|Texas Instruments Incorporated
|ADS890xB 20-Bit, High-Speed SAR ADCs With Integrated Reference Buffer, and
|Enhanced Performance Features
[IBIS Ver]   4.1
[File name]   ads890xb.ibs
[Date]   07/31/2018
[File Rev]   1.0
[Source]
| Texas Instruments Incorporated.
| Analog-eLab Design Center, HPA
| 12500 TI Blvd
| Dallas, TX -75243
[Notes]   Revision History:
| Rev 1.0: 07/31/2018
| - Initial version of the model
| - Model generated from simulations in SPECTRE
| - Warnings regarding combined Non-monotonicity of various models
|   have been reviewed and considered minor and can be ignored.
| - C_comp although listed in numerical order of value are
|   obtained from varying PVT conditions. For PVT conditions for
|   each specific value refer the buffer description under
|   respective [Model]. IBIS model user is responsible for using
|   appropriate C_comp to simulate for Signal Integrity.
[Disclaimer]
| This model is designed as an aid for customers of Texas Instruments.
| TI and its licensors and suppliers make no warranties, either expressed
| or implied, with respect to this  model, including the warranties of
| merchantability or fitness for a particular purpose. The model is
| provided solely on an "as is" basis. The entire risk as to its quality
| and performance is with the customer.
| This model is subject to change without notice. Texas Instruments
| Incorporated is not responsible for updating this model.
[Copyright]
(C) Copyright 2018 Texas Instruments Incorporated.All rights reserved.
|  Component ADS8900BRGER 24-pin VQFN - RGE package
|  Part # ADS8900BRGER
[Component]   ADS8900BRGER
[Manufacturer]  TI
[Package]   |24-pin VQFN - RGE package
|   typ   min   max
R_pkg   0.05   0.04   0.06
L_pkg   1.0nH   0.8nH   1.2nH
C_pkg   0.2pF   0.16pF   0.24pF
[Pin] signal_name model_name R_pin L_pin C_pin
1   CONVST   INPUT   NA   NA   NA
2   RSTZ   INPUT   NA   NA   NA
3   REFIN   NC   NA   NA   NA
4   REFM   NC   NA   NA   NA
5   REFBUFOUT   NC   NA   NA   NA
6   NC   NC   NA   NA   NA
7   REFBUFOUT   NC   NA   NA   NA
8   REFM   NC   NA   NA   NA
9   AINP   NC   NA   NA   NA
10   AINM   NC   NA   NA   NA
11   GND   GND   NA   NA   NA
12   RVDD   POWER   NA   NA   NA
13   DECAP   POWER   NA   NA   NA
14   DECAP   POWER   NA   NA   NA
15   GND   GND   NA   NA   NA
16   DVDD   POWER   NA   NA   NA
17   SDO-3   OUTPUT   NA   NA   NA
18   SDO-2   OUTPUT   NA   NA   NA
19   SDO-1   OUTPUT   NA   NA   NA
20   SDO-0   OUTPUT   NA   NA   NA
21   RVS   OUTPUT   NA   NA   NA
22   SDI   INPUT   NA   NA   NA
23   SCLK   INPUT   NA   NA   NA
24   CSZ   INPUT   NA   NA   NA
|  Component ADS8900BRGET 24-pin VQFN - RGE package
|  Part # ADS8900BRGET
[Component]   ADS8900BRGET
[Manufacturer]  TI
[Package]   |24-pin VQFN - RGE package
|   typ   min   max
R_pkg   0.05   0.04   0.06
L_pkg   1.0nH   0.8nH   1.2nH
C_pkg   0.2pF   0.16pF   0.24pF
[Pin] signal_name model_name R_pin L_pin C_pin
1   CONVST   INPUT   NA   NA   NA
2   RSTZ   INPUT   NA   NA   NA
3   REFIN   NC   NA   NA   NA
4   REFM   NC   NA   NA   NA
5   REFBUFOUT   NC   NA   NA   NA
6   NC   NC   NA   NA   NA
7   REFBUFOUT   NC   NA   NA   NA
8   REFM   NC   NA   NA   NA
9   AINP   NC   NA   NA   NA
10   AINM   NC   NA   NA   NA
11   GND   GND   NA   NA   NA
12   RVDD   POWER   NA   NA   NA
13   DECAP   POWER   NA   NA   NA
14   DECAP   POWER   NA   NA   NA
15   GND   GND   NA   NA   NA
16   DVDD   POWER   NA   NA   NA
17   SDO-3   OUTPUT   NA   NA   NA
18   SDO-2   OUTPUT   NA   NA   NA
19   SDO-1   OUTPUT   NA   NA   NA
20   SDO-0   OUTPUT   NA   NA   NA
21   RVS   OUTPUT   NA   NA   NA
22   SDI   INPUT   NA   NA   NA
23   SCLK   INPUT   NA   NA   NA
24   CSZ   INPUT   NA   NA   NA
|  Component ADS8902BRGER 24-pin VQFN - RGE package
|  Part # ADS8902BRGER
[Component]   ADS8902BRGER
[Manufacturer]  TI
[Package]   |24-pin VQFN - RGE package
|   typ   min   max
R_pkg   0.05   0.04   0.06
L_pkg   1.0nH   0.8nH   1.2nH
C_pkg   0.2pF   0.16pF   0.24pF
[Pin] signal_name model_name R_pin L_pin C_pin
1   CONVST   INPUT   NA   NA   NA
2   RSTZ   INPUT   NA   NA   NA
3   REFIN   NC   NA   NA   NA
4   REFM   NC   NA   NA   NA
5   REFBUFOUT   NC   NA   NA   NA
6   NC   NC   NA   NA   NA
7   REFBUFOUT   NC   NA   NA   NA
8   REFM   NC   NA   NA   NA
9   AINP   NC   NA   NA   NA
10   AINM   NC   NA   NA   NA
11   GND   GND   NA   NA   NA
12   RVDD   POWER   NA   NA   NA
13   DECAP   POWER   NA   NA   NA
14   DECAP   POWER   NA   NA   NA
15   GND   GND   NA   NA   NA
16   DVDD   POWER   NA   NA   NA
17   SDO-3   OUTPUT   NA   NA   NA
18   SDO-2   OUTPUT   NA   NA   NA
19   SDO-1   OUTPUT   NA   NA   NA
20   SDO-0   OUTPUT   NA   NA   NA
21   RVS   OUTPUT   NA   NA   NA
22   SDI   INPUT   NA   NA   NA
23   SCLK   INPUT   NA   NA   NA
24   CSZ   INPUT   NA   NA   NA
|  Component ADS8902BRGET 24-pin VQFN - RGE package
|  Part # ADS8902BRGET
[Component]   ADS8902BRGET
[Manufacturer]  TI
[Package]   |24-pin VQFN - RGE package
|   typ   min   max
R_pkg   0.05   0.04   0.06
L_pkg   1.0nH   0.8nH   1.2nH
C_pkg   0.2pF   0.16pF   0.24pF
[Pin] signal_name model_name R_pin L_pin C_pin
1   CONVST   INPUT   NA   NA   NA
2   RSTZ   INPUT   NA   NA   NA
3   REFIN   NC   NA   NA   NA
4   REFM   NC   NA   NA   NA
5   REFBUFOUT   NC   NA   NA   NA
6   NC   NC   NA   NA   NA
7   REFBUFOUT   NC   NA   NA   NA
8   REFM   NC   NA   NA   NA
9   AINP   NC   NA   NA   NA
10   AINM   NC   NA   NA   NA
11   GND   GND   NA   NA   NA
12   RVDD   POWER   NA   NA   NA
13   DECAP   POWER   NA   NA   NA
14   DECAP   POWER   NA   NA   NA
15   GND   GND   NA   NA   NA
16   DVDD   POWER   NA   NA   NA
17   SDO-3   OUTPUT   NA   NA   NA
18   SDO-2   OUTPUT   NA   NA   NA
19   SDO-1   OUTPUT   NA   NA   NA
20   SDO-0   OUTPUT   NA   NA   NA
21   RVS   OUTPUT   NA   NA   NA
22   SDI   INPUT   NA   NA   NA
23   SCLK   INPUT   NA   NA   NA
24   CSZ   INPUT   NA   NA   NA
|  Component ADS8904BRGER 24-pin VQFN - RGE package
|  Part # ADS8904BRGER
[Component]   ADS8904BRGER
[Manufacturer]  TI
[Package]   |24-pin VQFN - RGE package
|   typ   min   max
R_pkg   0.05   0.04   0.06
L_pkg   1.0nH   0.8nH   1.2nH
C_pkg   0.2pF   0.16pF   0.24pF
[Pin] signal_name model_name R_pin L_pin C_pin
1   CONVST   INPUT   NA   NA   NA
2   RSTZ   INPUT   NA   NA   NA
3   REFIN   NC   NA   NA   NA
4   REFM   NC   NA   NA   NA
5   REFBUFOUT   NC   NA   NA   NA
6   NC   NC   NA   NA   NA
7   REFBUFOUT   NC   NA   NA   NA
8   REFM   NC   NA   NA   NA
9   AINP   NC   NA   NA   NA
10   AINM   NC   NA   NA   NA
11   GND   GND   NA   NA   NA
12   RVDD   POWER   NA   NA   NA
13   DECAP   POWER   NA   NA   NA
14   DECAP   POWER   NA   NA   NA
15   GND   GND   NA   NA   NA
16   DVDD   POWER   NA   NA   NA
17   SDO-3   OUTPUT   NA   NA   NA
18   SDO-2   OUTPUT   NA   NA   NA
19   SDO-1   OUTPUT   NA   NA   NA
20   SDO-0   OUTPUT   NA   NA   NA
21   RVS   OUTPUT   NA   NA   NA
22   SDI   INPUT   NA   NA   NA
23   SCLK   INPUT   NA   NA   NA
24   CSZ   INPUT   NA   NA   NA
|  Component ADS8904BRGET 24-pin VQFN - RGE package
|  Part # ADS8904BRGET
[Component]   ADS8904BRGET
[Manufacturer]  TI
[Package]   |24-pin VQFN - RGE package
|   typ   min   max
R_pkg   0.05   0.04   0.06
L_pkg   1.0nH   0.8nH   1.2nH
C_pkg   0.2pF   0.16pF   0.24pF
[Pin] signal_name model_name R_pin L_pin C_pin
1   CONVST   INPUT   NA   NA   NA
2   RSTZ   INPUT   NA   NA   NA
3   REFIN   NC   NA   NA   NA
4   REFM   NC   NA   NA   NA
5   REFBUFOUT   NC   NA   NA   NA
6   NC   NC   NA   NA   NA
7   REFBUFOUT   NC   NA   NA   NA
8   REFM   NC   NA   NA   NA
9   AINP   NC   NA   NA   NA
10   AINM   NC   NA   NA   NA
11   GND   GND   NA   NA   NA
12   RVDD   POWER   NA   NA   NA
13   DECAP   POWER   NA   NA   NA
14   DECAP   POWER   NA   NA   NA
15   GND   GND   NA   NA   NA
16   DVDD   POWER   NA   NA   NA
17   SDO-3   OUTPUT   NA   NA   NA
18   SDO-2   OUTPUT   NA   NA   NA
19   SDO-1   OUTPUT   NA   NA   NA
20   SDO-0   OUTPUT   NA   NA   NA
21   RVS   OUTPUT   NA   NA   NA
22   SDI   INPUT   NA   NA   NA
23   SCLK   INPUT   NA   NA   NA
24   CSZ   INPUT   NA   NA   NA
| Models and submodels in the file (2): INPUT (Input), OUTPUT (3-state)
